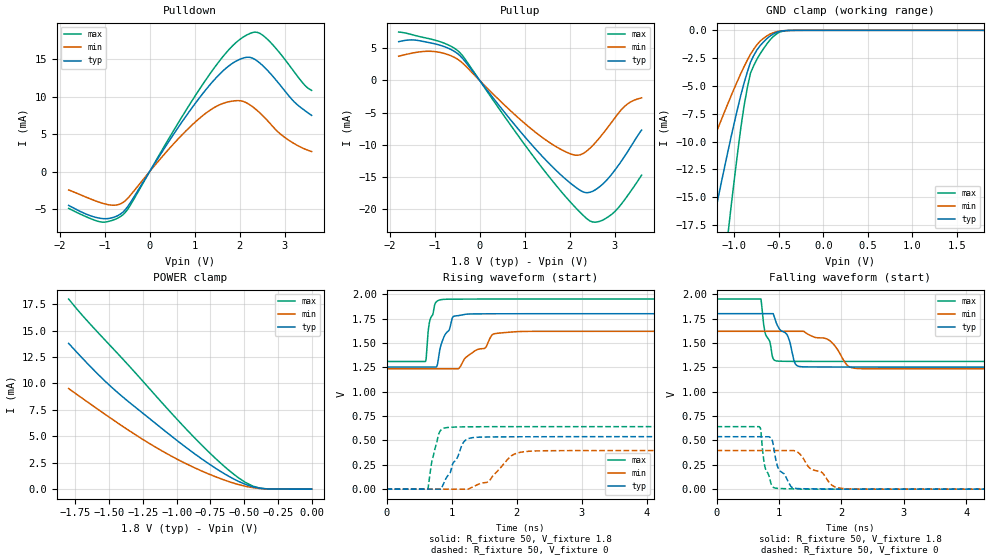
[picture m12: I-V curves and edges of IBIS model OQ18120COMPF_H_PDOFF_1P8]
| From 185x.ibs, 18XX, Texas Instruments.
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|   Model Cell OQ18120COMPF_H_PDOFF_1P8
|OQ18120COMPF_H_PDOFF_1P8
[Model]   OQ18120COMPF_H_PDOFF_1P8
Model_type   3-state
Polarity   Non-Inverting
Enable   Active-Low
Cref =  15pF
Rref =  100.0000M
Vref =  0V
Vmeas =  0.9
C_comp   3.022169p   2.248679p   3.342693p
[Temperature Range]   25   125   -40
[Voltage Range]   1.8   1.62   1.95
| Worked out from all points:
|   slope of the pulldown table from 0 to 0.27 V, typ, clamps not added: 105 ohm
|   slope of the pullup table from 0 to 0.27 V, typ, clamps not added: 110 ohm
|   GND clamp passes 1 mA (typ) near -0.67 V on its own axis
|   POWER clamp passes 1 mA (typ) near -0.58 V on its own axis
|   rising waveform, R_fixture 50, V_fixture 1.8: 20-80 % time 184ps typ, 410ps min, 101ps max; typ from 1.25 V to 1.8 V
|   rising waveform, R_fixture 50, V_fixture 0: 20-80 % time 234ps typ, 309ps min, 120ps max; typ from 0 V to 0.539 V
|   falling waveform, R_fixture 50, V_fixture 1.8: 20-80 % time 257ps typ, 284ps min, 142ps max; typ from 1.8 V to 1.25 V
|   falling waveform, R_fixture 50, V_fixture 0: 20-80 % time 209ps typ, 404ps min, 122ps max; typ from 0.539 V to 0 V
| Nom Voltages:
|   VBBNW=1.1, VDD=1.1, VDDS=1.8, ESD_BIASFET=0, ESD_VDDS=0, ESD_VSS=0,
|   VSS=0, VSSS=0
| Min Voltages:
|   VBBNW=0.99, VDD=0.99, VDDS=1.62, ESD_BIASFET=0, ESD_VDDS=0, ESD_VSS=0,
|   VSS=0, VSSS=0
| Max Voltages:
|   VBBNW=1.21, VDD=1.21, VDDS=1.95, ESD_BIASFET=0, ESD_VDDS=0, ESD_VSS=0,
|   VSS=0, VSSS=0
[POWER_clamp]
|   voltage   I(typ)   I(min)   I(max)
-1.8V     13.79mA    9.516mA    17.98mA
-1.691V   12.29mA    8.522mA    16.33mA
-1.582V   10.86mA    7.539mA    14.8mA
-1.364V   8.345mA    5.636mA    11.82mA
-1.145V   6.107mA    3.891mA    8.703mA
-981.8mV  4.451mA    2.74mA     6.401mA
-763.6mV  2.418mA    1.443mA    3.534mA
-600mV    1.12mA     659.7uA    1.647mA
-490.9mV  454.6uA    272.9uA    642.7uA
-436.4mV  225.3uA    141.7uA    291.2uA
-381.8mV  86.6uA     59.98uA    90.93uA
0V        312.2pA    762.9pA    3.032nA
[Pulldown]
|   voltage   I(typ)   I(min)   I(max)
-1.8V     -4.515mA   -2.451mA   -4.909mA
-1.036V   -6.278mA   -4.249mA   -6.752mA
-763.6mV  -6.024mA   -4.482mA   -6.361mA
-545.5mV  -5.116mA   -3.911mA   -5.476mA
545.5mV   5.097mA    3.788mA    5.6mA
1.2V      10.56mA    7.562mA    11.82mA
1.745V    14.03mA    9.297mA    16.16mA
2.182V    15.27mA    9.079mA    18.3mA
2.4V      14.72mA    8.101mA    18.57mA
2.564V    13.85mA    7.159mA    17.95mA
3V        10.8mA     4.573mA    15.01mA
3.6V      7.496mA    2.676mA    10.83mA
[Pullup]
|   voltage   I(typ)   I(min)   I(max)
-1.8V     6.014mA    3.756mA    7.497mA
-1.473V   6.279mA    4.274mA    7.043mA
-1.036V   5.74mA     4.497mA    6.327mA
-436.4mV  3.832mA    3.025mA    4.29mA
600mV     -5.351mA   -4.136mA   -6.059mA
1.309V    -11.14mA   -8.407mA   -12.83mA
1.964V    -15.62mA   -11.22mA   -18.44mA
2.291V    -17.26mA   -11.37mA   -20.85mA
2.564V    -16.99mA   -9.716mA   -21.98mA
2.891V    -14.92mA   -6.885mA   -20.99mA
3.218V    -11.81mA   -4.041mA   -18.54mA
3.6V      -7.699mA   -2.699mA   -14.69mA
[GND_clamp]
|   voltage   I(typ)   I(min)   I(max)
-1.8V     -40.54mA   -21.7mA    -74.86mA
-1.582V   -31.33mA   -17.07mA   -57.53mA
-1.255V   -17.92mA   -10.24mA   -32mA
-1.073V   -10.92mA   -6.597mA   -18.43mA
-1.036V   -9.578mA   -5.892mA   -15.84mA
-927.3mV  -5.833mA   -3.882mA   -8.768mA
-854.5mV  -3.75mA    -2.687mA   -5.167mA
-781.8mV  -2.256mA   -1.686mA   -3.165mA
-636.4mV  -765.4uA   -511.6uA   -1.245mA
-490.9mV  -89.46uA   -65.33uA   -151uA
-381.8mV  -7.537uA   -6.765uA   -11.19uA
1.8V      312.2pA    545.6nA    2.96nA
[Ramp]
| variable   typ   min   max
dV/dt_f 0.33782739/0.26393246n 0.23754504/0.32607515n 0.39708868/0.14315884n
dV/dt_r 0.33383655/0.24201034n 0.24427227/0.32732024n 0.40168159/0.1220998n
R_load = 50
[Rising Waveform]
R_fixture = 50
V_fixture = 1.8
V_fixture_min = 1.62
V_fixture_max = 1.95
|   time   V(typ)   V(min)   V(max)
0s        1.253V     1.235V     1.31V
600ps     1.253V     1.235V     1.31V
667.9ps   1.253V     1.235V     1.735V
773.8ps   1.261V     1.235V     1.927V
863.6ps   1.531V     1.235V     1.946V
1.036ns   1.773V     1.235V     1.949V
1.515ns   1.799V     1.449V     1.95V
1.634ns   1.799V     1.588V     1.95V
1.958ns   1.799V     1.615V     1.95V
11.2ns    1.8V       1.62V      1.95V
[Rising Waveform]
R_fixture = 50
V_fixture = 0
V_fixture_min = 0
V_fixture_max = 0
|   time   V(typ)   V(min)   V(max)
0s        0V         0V         0V
635ps     0V         0V         0V
693.9ps   0V         0V         276.3mV
802.9ps   0V         0V         567mV
959.3ps   151.9mV    0V         633.9mV
1.184ns   481.9mV    0V         639.1mV
1.391ns   532.4mV    44.31mV    640.4mV
1.93ns    537.2mV    346.9mV    641.1mV
2.229ns   537.9mV    390.6mV    641.2mV
11.23ns   539.1mV    396.9mV    641.8mV
[Falling Waveform]
R_fixture = 50
V_fixture = 1.8
V_fixture_min = 1.62
V_fixture_max = 1.95
|   time   V(typ)   V(min)   V(max)
0s        1.801V     1.62V      1.95V
711.6ps   1.801V     1.62V      1.95V
779.2ps   1.801V     1.62V      1.599V
979ps     1.674V     1.62V      1.314V
1.138ns   1.573V     1.62V      1.311V
1.26ns    1.287V     1.62V      1.311V
1.373ns   1.256V     1.62V      1.311V
1.803ns   1.253V     1.528V     1.31V
2.255ns   1.253V     1.238V     1.31V
11.2ns    1.252V     1.234V     1.31V
[Falling Waveform]
R_fixture = 50
V_fixture = 0
V_fixture_min = 0
V_fixture_max = 0
|   time   V(typ)   V(min)   V(max)
0s        538.5mV    396.6mV    641.3mV
694.6ps   538.5mV    396.6mV    634.5mV
779.6ps   538.5mV    396.6mV    215.9mV
887.7ps   507.4mV    396.6mV    32.95mV
971.9ps   242.1mV    396.6mV    8.347mV
1.227ns   14.16mV    396.6mV    2.926mV
1.691ns   2.461mV    169.3mV    0V
1.85ns    0V         39.97mV    0V
2.063ns   0V         4.781mV    0V
11.23ns   0V         0V         0V
